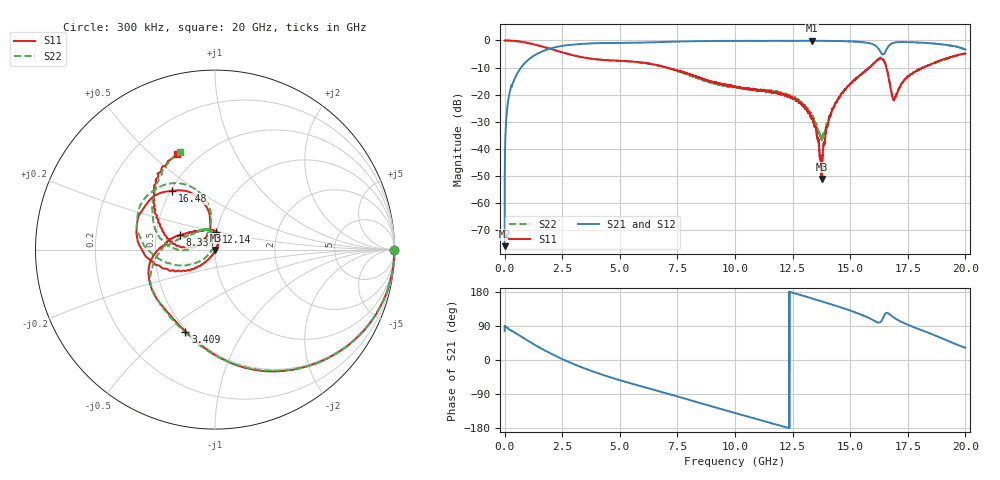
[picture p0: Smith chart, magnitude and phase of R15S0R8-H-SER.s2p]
!{R15S0R8}
!Johanson Technology Inc.
!www.johansontechnology.com
!Test Board Conditions:
!Substrate Type  RO4350B
!Substrate Thickness  20 mil
!Substrate Dk  3.66
!TL Type: GCPW
!TL Trace Width  34 mil
!TL Gap  10 mil
!Electrode orientation  Horizontal
!DUT TOPOLOGY	SERIES
!Mounting Pad LxW  26x52 mil
! Created Sat Feb  6 12:08:38 2021
# hz S ma R 50
! 2 Port Network Data from SP1.SP block
! freq  magS11  angS11  magS21  angS21  magS12  angS12  magS22  angS22
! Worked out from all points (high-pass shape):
!   20001 points, 300 kHz to 20 GHz, reference 50 ohm
!   highest |S21| = -0.11 dB at 13.36 GHz (marker M1); lowest = -76.0 dB at 300 kHz (marker M2)
!   |S21| within 3 dB of the highest: 1.936 GHz to 16.23 GHz (14.3 GHz wide, 157 % of centre); 16.59 GHz to 19.92 GHz (3.329 GHz wide, 18.2 % of centre)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
!   lowest |S11| = -51.2 dB at 13.77 GHz (marker M3), VSWR 1.01, Z = 50.2 - j0.167 ohm
!   |S11| at or under -10 dB: 7.019122 GHz to 7.019726 GHz (604.3 kHz wide, 0.00861 % of centre); 7.021 GHz to 15.83 GHz (8.813 GHz wide, 77.1 % of centre); 16.57 GHz to 18.21 GHz (1.638 GHz wide, 9.42 % of centre)
!   |S22| runs from -36.8 to 0.0 dB; largest |S21 - S12| = 0.018
!   S11 on the Smith chart (normalised r, x): 300 kHz: open; 3.409 GHz: 0.49, -0.58; 8.334 GHz: 0.66, +0.11; 12.14 GHz: 0.99, +0.19; 16.48 GHz: 0.51, +0.40; 20 GHz: 0.39, +0.61
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300000  0.9964 -0.1  0.0001589 76.9  0.0001791 69.9  0.9959 -0.2
1.013e8  0.9985 -4.3  0.05063 85.4  0.05088 85.4  0.9983 -4.4
1.363e8  0.9969 -5.8  0.06797 83.8  0.06835 83.9  0.9974 -5.8
5.233e8  0.9711 -20.4  0.2353 69.3  0.2358 69.4  0.9705 -20.4
1.6163e9  0.7768 -60.5  0.6232 29.5  0.6247 29.5  0.7758 -60.2
3.3343e9  0.4927 -108.1  0.8642 -19.0  0.8656 -19.0  0.4922 -109.5
3.4093e9  0.4861 -109.8  0.8685 -20.7  0.8688 -20.8  0.4861 -111.4
6.6673e9  0.3462 -174.2  0.93 -81.8  0.9312 -81.8  0.3425 -169.2
8.3343e9  0.2126 157.9  0.9697 -110.9  0.9712 -110.8  0.2038 162.7
1.00003e10  0.1407 133.2  0.9814 -139.8  0.9821 -139.8  0.1371 129.8
1.21433e10  0.0971 86.1  0.984 -176.3  0.9824 -176.4  0.1027 103.6
1.33343e10  0.03595 60.0  0.9844 162.7  0.9843 162.7  0.04001 96.8
1.33583e10  0.03623 61.6  0.9872 162.2  0.9832 162.3  0.0405 94.6
1.37733e10  0.002763 -37.1  0.9842 154.6  0.984 154.6  0.0146 149.0
1.40453e10  0.0297 -117.1  0.9795 149.5  0.981 149.5  0.03216 -148.7
1.45503e10  0.09155 -128.7  0.9737 139.8  0.973 139.7  0.09175 -140.6
1.58623e10  0.3224 -163.8  0.8857 109.5  0.8862 109.5  0.3224 -171.8
1.64753e10  0.4051 125.9  0.5657 117.7  0.5618 118.6  0.43 120.7
1.66673e10  0.206 99.1  0.7902 122.4  0.782 123.0  0.2178 96.6
1.69253e10  0.08286 147.8  0.9132 110.9  0.9121 111.2  0.0856 148.4
1.76883e10  0.2439 169.9  0.9263 88.2  0.9272 88.7  0.2455 176.7
2e10  0.5698 111.6  0.6782 32.2  0.6706 32.2  0.5766 109.6
